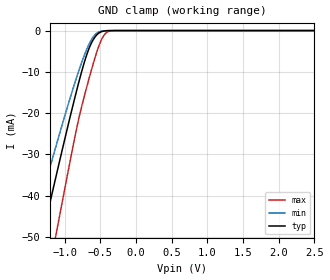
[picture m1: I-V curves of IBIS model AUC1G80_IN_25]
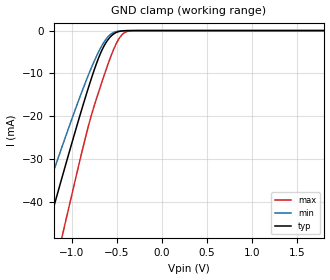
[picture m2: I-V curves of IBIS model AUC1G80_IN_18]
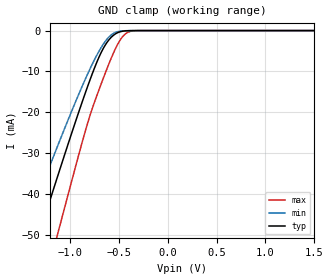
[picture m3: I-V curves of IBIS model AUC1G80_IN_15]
| TEXAS INSTRUMENTS INCORPORATED
| Standard Linear and Logic Group
| IBIS Model of SN74AUC1G80
| SINGLE POSITIVE-EDGE-TRIGGERED D-TYPE FLIP-FLOP
| This file contains package information for the following:
|  SOT 5-pin (DBV) package as [Component] AUC1G80_DBV
|  SOT 5-pin (DCK) package as [Component] AUC1G80_DCK
|  NanoStar WCSP 5-pin (YEA) package as [Component] AUC1G80_YEA
|  NanoFree WCSP 5-pin (YZA) package as [Component] AUC1G80_YZA
|  NanoStar WCSP 5-pin (YEP) package as [Component] AUC1G80_YEP
|  NanoFree WCSP 5-pin (YZP) package as [Component] AUC1G80_YZP
| This device can be powered at the following Vccs:
|  2.5 volt Vcc
|  1.8 volt Vcc
|  1.5 volt Vcc
|  1.2 volt Vcc
|  0.8 volt Vcc
| This file provides unique models under the [Model Selector] for each Vcc.
| For operation at a specific Vcc, select the appropriate model after each
| [Model Selector] keyword.
[IBIS Ver]   3.2
[Comment char]  |_char
[File Name]   sn74auc1g80.ibs
[File Rev]   1.1 | x_die
[Date]   October 08, 2003
[Source]   Data created from TI-SPICE simulations at TI-SLL.
[Notes]   The following is an IBIS list for the AUC1G80.
   Please contact sllibis@ti.com with questions and
   comments concerning SLL IBIS models.
   -The waveforms for the AUC1G80_OUT Pullup, and
   Pulldown are caused by the circuitry that helps reduce
   overshoot and undershoot in transmission lines (EMI).
   These waveforms are normal for this particular design.
   -End point warning due to AC and DC mismatch.
   -Power clamp data deleted as there is no power-clamp diode.
[Disclaimer] Property of Texas Instruments Incorporated.  Unauthorized
   reproduction and/or distribution is strictly prohibited.
   This product is protected under copyright law.
   Created  2002, (C) Copyright  2002, Texas Instruments
   Incorporated, All Rights Reserved
   UNLESS THERE IS A SIGNED, WRITTEN AGREEMENT TO THE
   CONTRARY, TEXAS INSTRUMENTS (TI) IS PROVIDING THE IBIS
   MODELS  AND WITHOUT ANY WARRANTY, EXPRESSED OR
   IMPLIED.  TI assumes no liability for:
   1) the accuracy of the IBIS models provided to your
   company;
   2) the proper functioning of these IBIS Models in your
   design or for any resulting applications; or
   3) infringement of patents, copyrights or intellectual
   property rights resulting from your use of these IBIS
   models.
   TI provides IBIS Models as a service to our customers.
   You and your company shall not distribute, sell or give
   these models to anyone else without prior written
   permission from TI.
   TI reserves the right to make changes to our products or
   to discontinue any semiconductor product or service
   without notice, and advises our customers to obtain the
   latest version of relevant information to verify, before
   placing orders, that the information being relied on is
   current.
   Please be aware that your receipt and use of the IBIS
   information provided shall serve as acceptance of these
   terms and conditions.  If you do not accept these terms,
   you should return or destroy the IBIS models and any
   other accompanying information immediately.
| Component AUC1G80_DBV 5-pin SOT
[Component]   AUC1G80_DBV
[Manufacturer]   Texas Instruments, Inc.
[Package]
|   typ   min   max
R_pkg   2.500e-02   2.100e-02   2.900e-02
L_pkg   1.529e-09   1.312e-09   1.906e-09
C_pkg   1.560e-13   1.100e-13   2.400e-13
[Pin]   signal_name   model_name   R_pin   L_pin   C_pin
1   D   AUC1G80_IN   2.100e-02   1.511e-09   1.440e-13
2   CLK   AUC1G80_IN   2.300e-02   1.312e-09   1.380e-13
3   GND   GND   2.900e-02   1.906e-09   2.400e-13
4   NQ   AUC1G80_OUT   2.600e-02   1.541e-09   1.500e-13
5   VCC   POWER   2.500e-02   1.374e-09   1.100e-13
| Component AUC1G80_DCK 5-pin SOT
[Component]   AUC1G80_DCK
[Manufacturer]   Texas Instruments, Inc.
[Package]
|   typ   min   max
R_pkg   2.000e-02   1.700e-02   2.500e-02
L_pkg   9.980e-10   8.810e-10   1.069e-09
C_pkg   1.460e-13   1.180e-13   2.050e-13
[Pin]   signal_name   model_name   R_pin   L_pin   C_pin
1   D   AUC1G80_IN   1.900e-02   1.069e-09   1.620e-13
2   CLK   AUC1G80_IN   1.800e-02   8.810e-10   1.210e-13
3   GND   GND   1.700e-02   1.031e-09   2.050e-13
4   YNQ   AUC1G80_OUT   2.000e-02   9.600e-10   1.240e-13
5   VCC   POWER   2.500e-02   1.049e-09   1.180e-13
| Component AUC1G80_YEA 5-pin NanoStar WCSP
[Component]   AUC1G80_YEA
[Manufacturer]   Texas Instruments, Inc.
[Package]
|   typ   min   max
R_pkg   0.001   0.001   0.001
L_pkg   0.021nH   0.021nH   0.021nH
C_pkg   0.046pF   0.045pF   0.047pF
[Pin]   signal_name   model_name   R_pin   L_pin   C_pin
1   D   AUC1G80_IN   0.001   0.021nH   0.046pF
2   CLK   AUC1G80_IN   0.001   0.021nH   0.047pF
3   GND   GND   0.001   0.021nH   0.046pF
4   NQ   AUC1G80_OUT   0.001   0.021nH   0.045pF
5   VCC   POWER   0.001   0.021nH   0.045pF
| Component AUC1G80_YZA 5-pin NanoFree WCSP
[Component]   AUC1G80_YZA
[Manufacturer]   Texas Instruments, Inc.
[Package]
|   typ   min   max
R_pkg   0.001   0.001   0.001
L_pkg   0.021nH   0.021nH   0.021nH
C_pkg   0.046pF   0.045pF   0.047pF
[Pin]   signal_name   model_name   R_pin   L_pin   C_pin
1   D   AUC1G80_IN   0.001   0.021nH   0.046pF
2   CLK   AUC1G80_IN   0.001   0.021nH   0.047pF
3   GND   GND   0.001   0.021nH   0.046pF
4   NQ   AUC1G80_OUT   0.001   0.021nH   0.045pF
5   VCC   POWER   0.001   0.021nH   0.045pF
| Component AUC1G80_YEP 5-pin NanoStar WCSP
[Component]   AUC1G80_YEP
[Manufacturer]   Texas Instruments, Inc.
[Package]
|   typ   min   max
R_pkg   0.001   0.001   0.001
L_pkg   0.021nH   0.021nH   0.021nH
C_pkg   0.046pF   0.045pF   0.047pF
[Pin]   signal_name   model_name   R_pin   L_pin   C_pin
1   D   AUC1G80_IN   0.001   0.021nH   0.046pF
2   CLK   AUC1G80_IN   0.001   0.021nH   0.047pF
3   GND   GND   0.001   0.021nH   0.046pF
4   NQ   AUC1G80_OUT   0.001   0.021nH   0.045pF
5   VCC   POWER   0.001   0.021nH   0.045pF
| Component AUC1G80_YZP 5-pin NanoFree WCSP
[Component]   AUC1G80_YZP
[Manufacturer]   Texas Instruments, Inc.
[Package]
|   typ   min   max
R_pkg   0.001   0.001   0.001
L_pkg   0.021nH   0.021nH   0.021nH
C_pkg   0.046pF   0.045pF   0.047pF
[Pin]   signal_name   model_name   R_pin   L_pin   C_pin
1   D   AUC1G80_IN   0.001   0.021nH   0.046pF
2   CLK   AUC1G80_IN   0.001   0.021nH   0.047pF
3   GND   GND   0.001   0.021nH   0.046pF
4   NQ   AUC1G80_OUT   0.001   0.021nH   0.045pF
5   VCC   POWER   0.001   0.021nH   0.045pF
| Model AUC1G80_IN
[Model Selector]   AUC1G80_IN
AUC1G80_IN_25   2.5 volt Vcc
AUC1G80_IN_18   1.8 volt Vcc
AUC1G80_IN_15   1.5 volt Vcc
AUC1G80_IN_12   1.2 volt Vcc
AUC1G80_IN_08   0.8 volt Vcc
| Model AUC1G80_OUT
[Model Selector]   AUC1G80_OUT
AUC1G80_OUT_25   2.5 volt Vcc
AUC1G80_OUT_18   1.8 volt Vcc
AUC1G80_OUT_15   1.5 volt Vcc
AUC1G80_OUT_12   1.2 volt Vcc
AUC1G80_OUT_08   0.8 volt Vcc
| Models and submodels in the file (10): AUC1G80_IN_25 (Input), AUC1G80_IN_18 (Input), AUC1G80_IN_15 (Input), AUC1G80_IN_12 (Input), AUC1G80_IN_08 (Input), AUC1G80_OUT_25 (Output), AUC1G80_OUT_18 (Output), AUC1G80_OUT_15 (Output), AUC1G80_OUT_12 (Output), AUC1G80_OUT_08 (Output)
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[Model]   AUC1G80_IN_25
Model_type  Input
Vinl=0.7
Vinh=1.7
| variable   typ   min   max
C_comp   2.46pF   1.97pF   2.84pF
[Temperature Range]   40   100   -40
| Ambient temperature   25   85   -40
[Voltage range]   2.5   2.3   2.7
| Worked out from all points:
|   GND clamp passes 1 mA (typ) near -0.55 V on its own axis
[GND Clamp]
| AUC1G80_IN_25
|   Voltage   I(typ)   I(min)   I(max)
-3.6V     -226.6mA   -190.3mA   -271.8mA
-1.455V   -60.71mA   -48.79mA   -79.87mA
-1.295V   -48.52mA   -38.74mA   -65.35mA
-1.105V   -34.25mA   -27.09mA   -48.1mA
-850mV    -15.85mA   -12.35mA   -25.34mA
-785mV    -11.51mA   -8.949mA   -20.15mA
-725mV    -7.81mA    -6.074mA   -16.01mA
-625mV    -3.071mA   -2.25mA    -9.633mA
-520mV    -618.6uA   -332uA     -3.783mA
-430mV    -73.2uA    -35.47uA   -776.9uA
-325mV    -3.339uA   -2.035uA   -30.74uA
2.5V      313.9pA    402pA      470.4pA
[Model]   AUC1G80_IN_18
Model_type  Input
Vinl=0.5775
Vinh=1.2675
| variable   typ   min   max
C_comp   2.53pF   2.06pF   2.87pF
[Temperature Range]   40   100   -40
| Ambient temperature   25   85   -40
[Voltage range]   1.8   1.65   1.95
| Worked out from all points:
|   GND clamp passes 1 mA (typ) near -0.55 V on its own axis
[GND Clamp]
| AUC1G80_IN_18
|   Voltage   I(typ)   I(min)   I(max)
-3.6V     -226.6mA   -190.3mA   -271.8mA
-1.435V   -59.19mA   -47.53mA   -78.05mA
-1.26V    -45.87mA   -36.57mA   -62.17mA
-1.105V   -34.25mA   -27.09mA   -48.1mA
-1.08V    -32.4mA    -25.59mA   -45.83mA
-810mV    -13.15mA   -10.23mA   -22.06mA
-685mV    -5.638mA   -4.364mA   -13.41mA
-565mV    -1.378mA   -858.8uA   -6.102mA
-490mV    -325.9uA   -162.9uA   -2.495mA
-425mV    -63.96uA   -31.11uA   -688.8uA
-300mV    -1.501uA   -1.001uA   -11.88uA
1.8V      203.2pA    298.4pA    235.5pA
[Model]   AUC1G80_IN_15
Model_type  Input
Vinl=0.49
Vinh=1.04
| variable   typ   min   max
C_comp   2.56pF   2.12pF   2.89pF
[Temperature Range]   40   100   -40
| Ambient temperature   25   85   -40
[Voltage range]   1.5   1.4   1.6
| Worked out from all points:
|   GND clamp passes 1 mA (typ) near -0.55 V on its own axis
[GND Clamp]
| AUC1G80_IN_15A
|   Voltage   I(typ)   I(min)   I(max)
-3.6V     -226.6mA   -190.3mA   -271.8mA
-1.465V   -61.48mA   -49.43mA   -80.77mA
-1.29V    -48.15mA   -38.43mA   -64.9mA
-1.13V    -36.11mA   -28.6mA    -50.37mA
-1.08V    -32.4mA    -25.59mA   -45.83mA
-815mV    -13.48mA   -10.49mA   -22.45mA
-695mV    -6.152mA   -4.773mA   -14.06mA
-575mV    -1.605mA   -1.034mA   -6.664mA
-500mV    -407.2uA   -207.5uA   -2.896mA
-435mV    -83.64uA   -40.42uA   -873uA
-310mV    -2.072uA   -1.331uA   -17.49uA
1.5V      165.9pA    259.7pA    172.1pA
